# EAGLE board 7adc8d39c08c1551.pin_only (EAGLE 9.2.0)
REV: B

Size 101.6 x 53.34 mm. Coordinates in mm from the lower left corner, seen from the top.
Outline: 97.54,53.34 99.06,51.82 99.06,40.39 101.6,37.85 101.6,5.08 99.06,2.54 99.06,1 arc-90 98.06,0 26.16,0 24.13,2.03 18.54,2.03 16.51,0 1,0 arc-90 0,1 0,15.37 0.89,16.26 0.89,25.91 0,26.8 0,34.16 0.51,34.67 0.51,41.53 0,42.04 0,52.34 arc-90 1,53.34 97.54,53.34
Copper layers (1*16): Top 0.035mm / dielectric 1.5mm / Bottom 0.035mm
Design rules "adafruit *": minimum track width 7mil, minimum drill 15.5mil, track to track 7mil, track to pad 7mil, pad to pad 7mil, via to via 7mil, smd to smd 7mil, copper to edge 10mil, drill to drill 8mil, minimum pad ring 10mil, minimum via ring 8mil, stop-mask expansion 2mil, vias tented up to drill 20mil, thermal gap 10mil
Holes 3.2 mm at 66.04,35.56 66.04,7.62 15.24,50.8 13.97,2.54 96.52,2.54 90.17,50.8

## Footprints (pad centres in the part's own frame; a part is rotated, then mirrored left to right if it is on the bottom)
1X08_OVALWAVE = drill 0.8 pad 1.5 long: 1 -8.89,0; 2 -6.35,0; 3 -3.81,0; 4 -1.27,0; 5 1.27,0; 6 3.81,0; 7 6.35,0; 8 8.89,0
0805-NO = smd 1.24 x 1.5: 1 -0.95,0; 2 0.95,0
0603-NO = smd 1.075 x 1: 1 -0.85,0; 2 0.85,0
SOD-123 = smd 1.4 x 1.4: A 1.85,0; C -1.85,0
R1206 = smd 1.6 x 1.803: 1 -1.422,0; 2 1.422,0
FIDUCIAL_1MM = smd 1 x 1: 1 0,0
SOLDERJUMPER_CLOSEDWIRE = smd 1.168 x 1.6: 1 -0.762,0; 2 0.762,0 | smd 0.635 x 0.203: WIRE 0,0
SOT23-5 = smd 0.69 x 0.99: 1 -0.95,-1.29; 2 0,-1.29; 3 0.95,-1.29; 4 0.95,1.3; 5 -0.95,1.3
2X03_ROUND_70MIL = drill 0.9 pad 1.778: 1 -2.54,-1.27; 2 -2.54,1.27; 3 0,-1.27; 4 0,1.27; 5 2.54,-1.27; 6 2.54,1.27
1X10_OVALWAVE = drill 0.8 pad 1.5 long: 1 -11.43,0; 2 -8.89,0; 3 -6.35,0; 4 -3.81,0; 5 -1.27,0; 6 1.27,0; 7 3.81,0; 8 6.35,0; 9 8.89,0; 10 11.43,0
1X01_ROUND = drill 1 pad 1.676: 1 0,0
2X18_THICKWAVE = drill 0.85 pad 1.778 octagon: 1 -21.59,-1.27; 2 -21.59,1.27; 3 -19.05,-1.27; 4 -19.05,1.27; 5 -16.51,-1.27; 6 -16.51,1.27; 7 -13.97,-1.27; 8 -13.97,1.27; 9 -11.43,-1.27; 10 -11.43,1.27; 11 -8.89,-1.27; 12 -8.89,1.27; 13 -6.35,-1.27; 14 -6.35,1.27; 15 -3.81,-1.27; 16 -3.81,1.27; 17 -1.27,-1.27; 18 -1.27,1.27; 19 1.27,-1.27; 20 1.27,1.27; 21 3.81,-1.27; 22 3.81,1.27; 23 6.35,-1.27; 24 6.35,1.27; 25 8.89,-1.27; 26 8.89,1.27; 27 11.43,-1.27; 28 11.43,1.27; 29 13.97,-1.27; 30 13.97,1.27; 31 16.51,-1.27; 32 16.51,1.27; 33 19.05,-1.27; 34 19.05,1.27; 35 21.59,-1.27; 36 21.59,1.27
CHIPLED_0805_NOOUTLINE = smd 1.2 x 1.2: A 0,-1.05; C 0,1.05
INDUCTOR_1007 = smd 1.016 x 2.2: P$1 -1.127,0; P$2 1.127,0
LED3535 = smd 1 x 0.85: 1 -1.75,0.875; 2 -1.75,-0.875; 3 1.75,-0.875; 4 1.75,0.875
PANASONIC_D = smd 3.556 x 1.4: + 2.654,0; - -2.654,0
RESPACK_4X0603 = smd 0.45 x 0.9: 1 -1.3,-0.85; 2 -0.4,-0.85; 3 0.4,-0.85; 4 1.3,-0.85; 5 1.3,0.85; 6 0.4,0.85; 7 -0.4,0.85; 8 -1.3,0.85
EVQ-Q2_SMALLER = smd 2 x 1.2: A -3.1,-2; A' 3.1,-2; B -3.1,2; B' 3.1,2
SPDT_SMT_SSSS811101 = smd 0.7 x 1.5: A -2.25,1.75; B 0.75,1.75; C 2.25,1.75 | smd 1 x 0.8: SUP1 -3.65,1.1; SUP2 -3.65,-1.1; SUP3 3.65,1.1; SUP4 3.65,-1.1 | hole 0.9: -1.5,0; 1.5,0
SOT-23 = smd 0.787 x 0.889: 1 0.025,-1.016; 2 -0.94,1.016; 3 0.991,1.016
SOT223-R = smd 1.3 x 1.3: 1 -2.3,-3.05; 2 0,-3.05; 3 2.3,-3.05 | smd 3.6 x 1.3: 4 0,3.05
SOT23-DBV = smd 0.55 x 1.2: 1 -0.95,-1.3; 2 0,-1.3; 3 0.95,-1.3; 4 0.95,1.3; 5 -0.95,1.3
SOIC8_208MIL = smd 0.6 x 2.2: 1 -1.905,-3.315; 2 -0.635,-3.315; 3 0.635,-3.315; 4 1.905,-3.315; 5 1.905,3.315; 6 0.635,3.315; 7 -0.635,3.315; 8 -1.905,3.315
SQFP-S-14X14-128 = smd 0.2 x 1.6: 1 -6.2,-7.6; 2 -5.8,-7.6; 3 -5.4,-7.6; 4 -5,-7.6; 5 -4.6,-7.6; 6 -4.2,-7.6; 7 -3.8,-7.6; 8 -3.4,-7.6; 9 -3,-7.6; 10 -2.6,-7.6; 11 -2.2,-7.6; 12 -1.8,-7.6; 13 -1.4,-7.6; 14 -1,-7.6; 15 -0.6,-7.6; 16 -0.2,-7.6; 17 0.2,-7.6; 18 0.6,-7.6; 19 1,-7.6; 20 1.4,-7.6; 21 1.8,-7.6; 22 2.2,-7.6; 23 2.6,-7.6; 24 3,-7.6; 25 3.4,-7.6; 26 3.8,-7.6; 27 4.2,-7.6; 28 4.6,-7.6; 29 5,-7.6; 30 5.4,-7.6; 31 5.8,-7.6; 32 6.2,-7.6; 65 6.2,7.6; 66 5.8,7.6; 67 5.4,7.6; 68 5,7.6; 69 4.6,7.6; 70 4.2,7.6; 71 3.8,7.6; 72 3.4,7.6; 73 3,7.6; 74 2.6,7.6; 75 2.2,7.6; 76 1.8,7.6; 77 1.4,7.6; 78 1,7.6; 79 0.6,7.6; 80 0.2,7.6; 81 -0.2,7.6; 82 -0.6,7.6; 83 -1,7.6; 84 -1.4,7.6; 85 -1.8,7.6; 86 -2.2,7.6; 87 -2.6,7.6; 88 -3,7.6; 89 -3.4,7.6; 90 -3.8,7.6; 91 -4.2,7.6; 92 -4.6,7.6; 93 -5,7.6; 94 -5.4,7.6; 95 -5.8,7.6; 96 -6.2,7.6 | smd 1.6 x 0.2: 33 7.6,-6.2; 34 7.6,-5.8; 35 7.6,-5.4; 36 7.6,-5; 37 7.6,-4.6; 38 7.6,-4.2; 39 7.6,-3.8; 40 7.6,-3.4; 41 7.6,-3; 42 7.6,-2.6; 43 7.6,-2.2; 44 7.6,-1.8; 45 7.6,-1.4; 46 7.6,-1; 47 7.6,-0.6; 48 7.6,-0.2; 49 7.6,0.2; 50 7.6,0.6; 51 7.6,1; 52 7.6,1.4; 53 7.6,1.8; 54 7.6,2.2; 55 7.6,2.6; 56 7.6,3; 57 7.6,3.4; 58 7.6,3.8; 59 7.6,4.2; 60 7.6,4.6; 61 7.6,5; 62 7.6,5.4; 63 7.6,5.8; 64 7.6,6.2; 97 -7.6,6.2; 98 -7.6,5.8; 99 -7.6,5.4; 100 -7.6,5; 101 -7.6,4.6; 102 -7.6,4.2; 103 -7.6,3.8; 104 -7.6,3.4; 105 -7.6,3; 106 -7.6,2.6; 107 -7.6,2.2; 108 -7.6,1.8; 109 -7.6,1.4; 110 -7.6,1; 111 -7.6,0.6; 112 -7.6,0.2; 113 -7.6,-0.2; 114 -7.6,-0.6; 115 -7.6,-1; 116 -7.6,-1.4; 117 -7.6,-1.8; 118 -7.6,-2.2; 119 -7.6,-2.6; 120 -7.6,-3; 121 -7.6,-3.4; 122 -7.6,-3.8; 123 -7.6,-4.2; 124 -7.6,-4.6; 125 -7.6,-5; 126 -7.6,-5.4; 127 -7.6,-5.8; 128 -7.6,-6.2
MICROSD = smd 0.7 x 1.5: 1 9,-10.64; 2 7.9,-10.24; 3 6.8,-10.64; 4 5.7,-11.04; 5 4.6,-10.64; 6 3.5,-11.04; 7 2.4,-10.64; 8 1.3,-10.64 | smd 1.8 x 1.4: CD1 2,-0.44; CD2 8,-0.44 | smd 1.4 x 1.9: MT1 0.4,-13.54; MT2 13.6,-14.44
2X05_1.27MM_BOX_POSTS = smd 0.76 x 2.6: 1 -2.54,-2.15; 2 -2.54,2.15; 3 -1.27,-2.15; 4 -1.27,2.15; 5 0,-2.15; 6 0,2.15; 7 1.27,-2.15; 8 1.27,2.15; 9 2.54,-2.15; 10 2.54,2.15 | hole 1: -1.905,0; 1.905,0
4UCONN_20329_V2 = smd 1 x 2: BASE@1 -0.75,-2; BASE@2 0.75,-2 | smd 0.4 x 1.35: D+ 0,0.775; D- -0.65,0.775; GND 1.3,0.775; ID 0.65,0.775; VBUS -1.3,0.775 | drill 0.8 pad 1.143 offset: SPRT@1 -3.3,0.9; SPRT@2 3.3,0.9 | drill 0.9 pad 2.413 square: SPRT@3 -3.6,-1.9; SPRT@4 3.6,-1.9 | hole 0.7: -1.95,0; 1.95,0
XTAL3215 = smd 1.1 x 1.9: P$1 1.2,0; P$2 -1.2,0
DCJACK_2MM_PTH = drill 0.9 pad 2.7 long: GND 7.35,0; GNDBREAK 10.75,-4.8; PWR 13.6,0

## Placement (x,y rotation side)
ANALOGH  20610  [1X08_OVALWAVE]  82.55,2.54 0 top
ANALOGL  20610  [1X08_OVALWAVE]  59.69,2.54 0 top
C1  10uF  [0805-NO]  29.09,23.98 270 top
C2  10uF  [0805-NO]  33.27,9.78 180 top
C3  10uF  [0805-NO]  34.54,14.1 180 top
C4  .1u  [0603-NO]  46.23,11.51 270 top
C5  22pF  [0603-NO]  42.42,12.06 90 top
C6  .1u  [0603-NO]  33.17,16.8 270 top
C7  22pF  [0603-NO]  41.53,15.11 0 top
C8  .1u  [0603-NO]  31.67,22.5 180 top
C9  1uF  [0603-NO]  28.34,27.14 180 top
C10  .1u  [0603-NO]  39.98,43.3 270 top
C11  .1u  [0603-NO]  35.38,24.53 45 top
C12  0.1uF  [0603-NO]  29.34,19.3 0 top
C13  0.1uF  [0603-NO]  34.54,12.32 0 top
C14  .1u  [0603-NO]  57.6,17.17 135 top
C15  .1u  [0603-NO]  47.75,11.4 90 top
C16  .1u  [0603-NO]  39.32,37.06 0 top
C17  0.1uF  [0603-NO]  14.35,45.49 90 top
C18  .1u  [0603-NO]  42.19,43.26 270 top
C19  .1u  [0603-NO]  57.15,38.61 270 top
C20  .1u  [0603-NO]  65.86,23.06 180 top
C21  .1u  [0603-NO]  58.95,29.64 0 top
C22  .1u  [0603-NO]  36.83,29.72 0 top
C23  .1u  [0603-NO]  44.07,11.53 90 top
C24  .1u  [0603-NO]  57.28,15.24 135 top
C25  .1u  [0603-NO]  68.83,29.74 270 top
D1  MBR120  [SOD-123]  13,8.48 90 top
F2  500mA  [R1206]  9.4,34.04 0 top
FB2  FERRITE  [0805-NO]  1.78,44.83 270 top
FD1  FIDUCIAL_1MM  [FIDUCIAL_1MM]  1.14,49.15 0 top
FD2  FIDUCIAL_1MM  [FIDUCIAL_1MM]  99.18,4.55 0 top
FD3  FIDUCIAL_1MM  [FIDUCIAL_1MM]  1.82,1.89 0 top
FD4  FIDUCIAL_1MM  [FIDUCIAL_1MM]  39.12,19.68 0 top
FD5  FIDUCIAL_1MM  [FIDUCIAL_1MM]  54.61,39.12 0 top
GROUND1  [SOLDERJUMPER_CLOSEDWIRE]  7.11,44.7 180 bottom
IC3  74LVC1G125D  [SOT23-5]  20.37,29.79 180 top
ICSP  3x2 M  [2X03_ROUND_70MIL]  64.9,27.94 270 top
IOH  20611  [1X10_OVALWAVE]  30.23,50.8 0 top
IOL  20610  [1X08_OVALWAVE]  54.61,50.8 0 top
JP1  [1X01_ROUND]  15.49,9.91 0 top
JP2  [2X18_THICKWAVE]  95.25,29.21 270 top
L  RED  [CHIPLED_0805_NOOUTLINE]  8.76,29.97 0 top
L1  10uH  [INDUCTOR_1007]  31.98,24.79 0 top
LED1  WS2812B3535  [LED3535]  11.3,41.15 180 top
ON  GREEN  [CHIPLED_0805_NOOUTLINE]  2.16,29.97 180 top
PC1  47uF/25V  [PANASONIC_D]  22.48,19.66 0 top
PC2  47uF+/6.3V+  [PANASONIC_D]  28.85,13.46 270 top
POWER  20610  [1X08_OVALWAVE]  36.83,2.54 0 top
R1  100K  [RESPACK_4X0603]  24.64,26.67 90 top
R2  1K  [RESPACK_4X0603]  12.83,30.23 180 top
R3  10K  [0603-NO]  16.02,45.48 90 top
R4  1K  [0603-NO]  87.38,11.81 90 top
R5  10K  [0603-NO]  71.25,27.18 90 top
R7  10K  [0603-NO]  14.48,12.06 180 top
R11  330R  [0603-NO]  21.13,33.3 0 top
RESET  EVQQ 6mm  [EVQ-Q2_SMALLER]  6.35,49.4 180 top
RXLED  YELLOW  [CHIPLED_0805_NOOUTLINE]  6.48,29.97 180 top
SJ1  AREF_3V  [SOLDERJUMPER_CLOSEDWIRE]  45.47,10.92 0 bottom
SW1  [SPDT_SMT_SSSS811101]  21.34,3.81 0 top
T2  DMP3098L-7  [SOT-23]  16.13,7.37 90 top
TR1  DMP3098L-7  [SOT-23]  19.35,25.65 0 top
TXLED  YELLOW  [CHIPLED_0805_NOOUTLINE]  4.32,29.97 180 top
U1  NCP1117ST50T3G  [SOT223-R]  21.13,12.22 90 top
U2  AP2112K-3.3  [SOT23-DBV]  36.32,16.76 90 top
U3  GD25Q64  [SOIC8_208MIL]  74.55,26.92 0 top
U$1  SAMD51PXXA  [SQFP-S-14X14-128]  48.26,27.94 0 top
U$23  [GRANDCENTRAL_REVB-BOT]  101.6,0 0 bottom
U$30  [GRANDCENTRAL_REVB_TOP]  0,0 0 top
UART  20610  [1X08_OVALWAVE]  77.47,50.8 0 top
X1  microsd  [MICROSD]  17.02,27.18 270 top
X2  2x5 0.05" SWD  [2X05_1.27MM_BOX_POSTS]  82.42,14.86 90 top
X3  20329  [4UCONN_20329_V2]  4.32,38.1 270 top
X4  32.768  [XTAL3215]  40.51,12.45 270 top
X5  2.1mm  [DCJACK_2MM_PTH]  -3.3,7.75 0 top

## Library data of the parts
ANALOGH ANALOGL C1-C25 D1 FB2 GROUND1 ICSP IOH IOL JP1 JP2 L L1 LED1 ON PC1 PC2 POWER R1-R5 R7 R11 RESET RXLED SJ1 SW1 TXLED U1 U3 U$1 UART X1-X3 X5 = microbuilder
F2 = adafruit
FD1-FD5 = microbuilder; BOM: EXCLUDE
IC3 = 74xx-little-de
T2 = zetex; OC_FARNELL: unknown; OC_NEWARK: unknown
TR1 = Transistors; CASE: SOT23; MONTHLY_USAGE: _____; PART_NUMBER: PMV48XP; PRICE: _____; SUPPLIER: _____; TYPE: Transistor
U2 = SmartPrj
U$23 U$30 = metro_silks
X4 = adafruit2

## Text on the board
tNames: 1 | 1 | DIGITAL
214bmp: D:/SmartProjects/Snc/a4_bn_logo2.bmp

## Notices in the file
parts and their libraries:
microbuilder: This work is placed in the public domain, and may be freely used for commercial and non-commercial work with the following conditions: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
